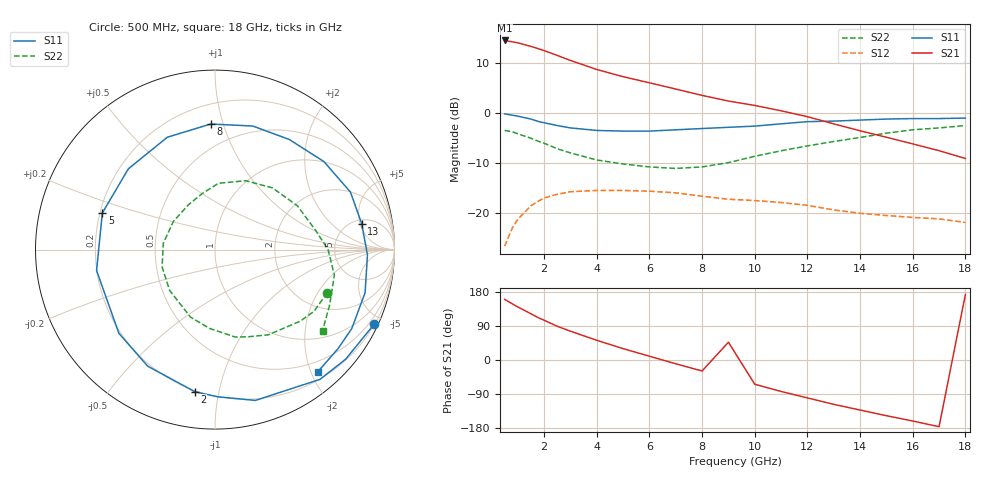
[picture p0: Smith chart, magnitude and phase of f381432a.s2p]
!ATF-38143
!S-PARAMETERS at Vds=2V  Id=5mA.  LAST UPDATED 20-10-99
# ghz s ma r 50
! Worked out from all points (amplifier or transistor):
!   23 points, 500 MHz to 18 GHz, reference 50 ohm
!   highest |S21| = 14.5 dB at 500 MHz (marker M1)
!   |S21| within 3 dB of that: start of sweep to 2.508 GHz
!   unconditionally stable (mu >= 1): 7.778 GHz to end of sweep
!   at 1.5 GHz: K = 0.21, MSG = 15.9 dB, |S12| = -18.5 dB
!   at 7 GHz: K = 0.88, MSG = 10.3 dB, |S12| = -15.9 dB
!   at 18 GHz: K = 1.83, MAG = 1.1 dB, |S12| = -21.8 dB
!   lowest NFmin = 0.18 dB at 500 MHz
!   S11 on the Smith chart (normalised r, x): 500 MHz: 0.22, -4.50; 2 GHz: 0.19, -0.85; 5 GHz: 0.21, +0.15; 8 GHz: 0.33, +0.91; 13 GHz: 5.75, +5.33; 18 GHz: 0.32, -2.10
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0.5  0.98 -25.0  5.289 160.0  0.047 73.0  0.67 -21.0
0.8  0.95 -40.0  5.122 148.0  0.072 63.0  0.65 -32.0
1  0.93 -51.0  5.01 140.0  0.087 56.0  0.62 -40.0
1.5  0.87 -75.0  4.613 122.0  0.119 41.0  0.56 -58.0
1.8  0.82 -89.0  4.362 111.0  0.133 33.0  0.52 -69.0
2  0.8 -98.0  4.192 105.0  0.142 28.0  0.5 -77.0
2.5  0.75 -120.0  3.751 89.0  0.155 16.0  0.44 -94.0
3  0.71 -139.0  3.342 76.0  0.164 5.0  0.4 -110.0
4  0.67 -170.0  2.716 52.0  0.169 -12.0  0.34 -138.0
5  0.66 162.0  2.302 30.0  0.169 -27.0  0.31 -162.0
6  0.66 137.0  2 10.0  0.166 -41.0  0.29 173.0
7  0.68 113.0  1.734 -10.0  0.16 -55.0  0.28 146.0
8  0.7 92.0  1.498 -29.0  0.148 -67.0  0.29 121.0
9  0.72 73.0  1.316 47.0  0.138 -77.0  0.32 103.0
10  0.74 56.0  1.19 -64.0  0.134 -86.0  0.37 87.0
11  0.78 39.0  1.052 -83.0  0.128 -97.0  0.42 66.0
12  0.82 23.0  0.919 -100.0  0.12 -106.0  0.47 47.0
13  0.83 10.0  0.779 -117.0  0.108 -115.0  0.52 28.0
15  0.87 -16.0  0.573 -147.0  0.095 -129.0  0.63 0.0
16  0.88 -30.0  0.492 -161.0  0.091 -136.0  0.68 -12.0
17  0.88 -39.0  0.421 -176.0  0.088 -145.0  0.71 -26.0
18  0.89 -50.0  0.352 173.0  0.081 -151.0  0.75 -37.0
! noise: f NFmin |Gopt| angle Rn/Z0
0.5  0.18  0.69  14  0.25
0.9  0.21  0.69  26  0.23
1.5  0.26  0.68  44  0.2
1.8  0.29  0.66  59  0.17
2.5  0.4  0.62  80  0.14
3  0.48  0.59  98  0.11
5  0.7  0.49  163  0.04
6  0.84  0.51  -169  0.04
8  1.12  0.54  -111  0.2
10  1.38  0.62  -68  0.6
